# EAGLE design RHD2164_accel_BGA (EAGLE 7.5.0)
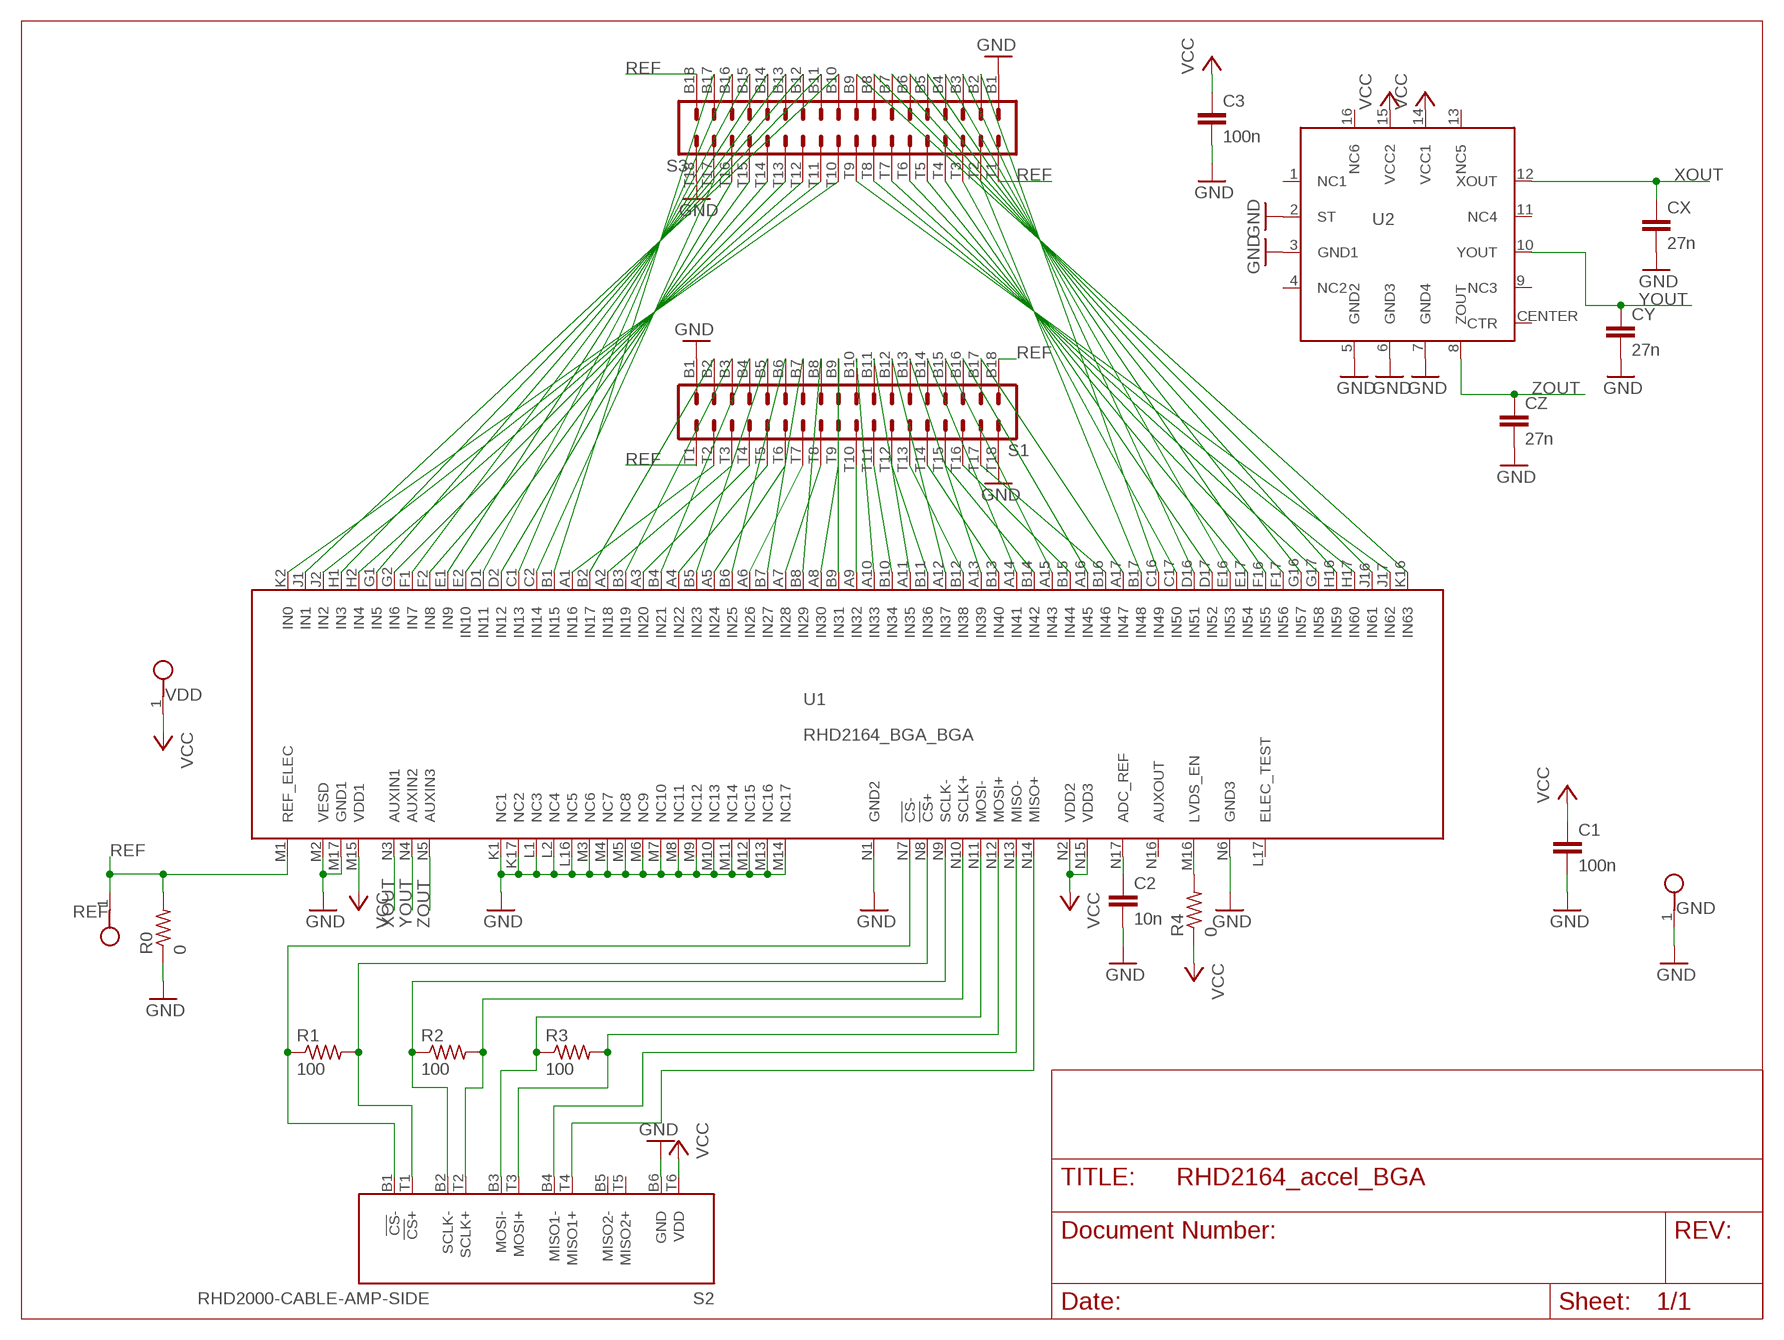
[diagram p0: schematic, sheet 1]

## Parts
C1  100n  C_0402  [0402]
C2  10n  C_0201  [0201]
C3  100n  C_0402  [0402]
CX  27n  C_0402  [0402]
CY  27n  C_0402  [0402]
CZ  27n  C_0402  [0402]
GND  TESTPOINT_SMALL  [TESTPOINT_SMALL]
R0  0  R_0402  [0402]
R1  100  R_0201  [0201]
R2  100  R_0201  [0201]
R3  100  R_0201  [0201]
R4  0  R_0402  [0402]
REF  TESTPOINT_SMALL  [TESTPOINT_SMALL]
S1  OMNETICS_A79025  [OMNETICS_A79025]
S2  RHD2000-CABLE-AMP-SIDE  [OMNETICS_PZN-12-AA]
S3  OMNETICS_A79025  [OMNETICS_A79025]
U1  RHD2164_BGA_BGA  [BGA104_9X7]
U2  ADXL335_IDAX  [ADXL335_IDAX]
VDD  TESTPOINT_SMALL  [TESTPOINT_SMALL]

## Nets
GND [thick]: C1.2 C2.2 C3.2 CX.2 CY.2 CZ.2 GND.1 R0.1 S1.B1 S1.T18 S2.B6(GND) S3.B1 S3.T18 U1.K1(NC1) U1.K17(NC2) U1.L1(NC3) U1.L2(NC4) U1.L16(NC5) U1.M2(VESD) U1.M3(NC6) U1.M4(NC7) U1.M5(NC8) U1.M6(NC9) U1.M7(NC10) U1.M8(NC11) U1.M9(NC12) U1.M10(NC13) U1.M11(NC14) U1.M12(NC15) U1.M13(NC16) U1.M14(NC17) U1.M17(GND1) U1.N1(GND2) U1.N6(GND3) U2.2(ST) U2.3(GND1) U2.5(GND2) U2.6(GND3) U2.7(GND4)
N$1: C2.1 U1.N17(ADC_REF)
N$2: S1.T2 U1.A1(IN16)
N$3: S1.B2 U1.B2(IN17)
N$4: S1.T3 U1.A2(IN18)
N$5: S1.B3 U1.B3(IN19)
N$6: S1.T4 U1.A3(IN20)
N$7: S1.B4 U1.B4(IN21)
N$8: S1.T5 U1.A4(IN22)
N$9: S1.B5 U1.B5(IN23)
N$10: S1.T6 U1.A5(IN24)
N$11: R1.1 S2.B1(!CS!-) U1.N7(!CS!-)
N$12: S1.B6 U1.B6(IN25)
N$13: S1.T7 U1.A6(IN26)
N$14: S1.B7 U1.B7(IN27)
N$15: S1.T8 U1.A7(IN28)
N$16: S1.B8 U1.B8(IN29)
N$17: S1.T9 U1.A8(IN30)
N$18: S1.B9 U1.B9(IN31)
N$19: S1.T10 U1.A9(IN32)
N$20: S1.B10 U1.A10(IN33)
N$21: S1.T11 U1.B10(IN34)
N$22: S1.B11 U1.A11(IN35)
N$23: S1.T12 U1.B11(IN36)
N$24: S1.B12 U1.A12(IN37)
N$25: S1.T13 U1.B12(IN38)
N$26: S1.B13 U1.A13(IN39)
N$27: S1.T14 U1.B13(IN40)
N$28: S1.B14 U1.A14(IN41)
N$29: S1.T15 U1.B14(IN42)
N$30: S1.B15 U1.A15(IN43)
N$31: S1.T16 U1.B15(IN44)
N$32: S1.B16 U1.A16(IN45)
N$33: S1.T17 U1.B16(IN46)
N$34: S1.B17 U1.A17(IN47)
N$35: R1.2 S2.T1(!CS!+) U1.N8(!CS!+)
N$36: R2.1 S2.B2(SCLK-) U1.N9(SCLK-)
N$37: R2.2 S2.T2(SCLK+) U1.N10(SCLK+)
N$38: R3.1 S2.B3(MOSI-) U1.N11(MOSI-)
N$39: R3.2 S2.T3(MOSI+) U1.N12(MOSI+)
N$40: S2.B4(MISO1-) U1.N13(MISO-)
N$41: S3.B17 U1.B1(IN15)
N$42: R4.2 U1.M16(LVDS_EN)
N$43: S3.T17 U1.C2(IN14)
N$44: S3.B16 U1.C1(IN13)
N$45: S3.T16 U1.D2(IN12)
N$46: S3.B15 U1.D1(IN11)
N$47: S3.T15 U1.E2(IN10)
N$48: S3.B14 U1.E1(IN9)
N$49: S3.T14 U1.F2(IN8)
N$50: S3.B13 U1.F1(IN7)
N$51: S3.T13 U1.G2(IN6)
N$52: S3.B12 U1.G1(IN5)
N$53: S3.T12 U1.H2(IN4)
N$54: S3.B11 U1.H1(IN3)
N$55: S3.T11 U1.J2(IN2)
N$56: S3.B10 U1.J1(IN1)
N$57: S3.T10 U1.K2(IN0)
N$58: S3.T2 U1.B17(IN48)
N$59: S3.B2 U1.C16(IN49)
N$60: S3.T3 U1.C17(IN50)
N$61: S3.B3 U1.D16(IN51)
N$62: S3.T4 U1.D17(IN52)
N$63: S3.B4 U1.E16(IN53)
N$64: S3.T5 U1.E17(IN54)
N$65: S3.B5 U1.F16(IN55)
N$66: S3.T6 U1.F17(IN56)
N$67: S3.B6 U1.G16(IN57)
N$68: S3.T7 U1.G17(IN58)
N$69: S3.B7 U1.H16(IN59)
N$70: S3.T8 U1.H17(IN60)
N$71: S3.B8 U1.J16(IN61)
N$72: S3.T9 U1.J17(IN62)
N$73: S3.B9 U1.K16(IN63)
N$74: S2.T4(MISO1+) U1.N14(MISO+)
REF [thick]: R0.2 REF.1 S1.B18 S1.T1 S3.B18 S3.T1 U1.M1(REF_ELEC)
VCC [thick]: C1.1 C3.1 R4.1 S2.T6(VDD) U1.M15(VDD1) U1.N2(VDD2) U1.N15(VDD3) U2.14(VCC1) U2.15(VCC2) VDD.1
XOUT: CX.1 U1.N3(AUXIN1) U2.12(XOUT)
YOUT: CY.1 U1.N4(AUXIN2) U2.10(YOUT)
ZOUT: CZ.1 U1.N5(AUXIN3) U2.8(ZOUT)
Unconnected: S2.B5(MISO2-) S2.T5(MISO2+) U1.L17(ELEC_TEST) U1.N16(AUXOUT) U2.1(NC1) U2.4(NC2) U2.9(NC3) U2.11(NC4) U2.13(NC5) U2.16(NC6) U2.CENTER(CTR)

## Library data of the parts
C1-C3 CX CY CZ = RHD2000_eval_board:C: Capacitor
GND REF VDD = RHD2000_eval_board:TESTPOINT: PCB Test Point
R0 R1-R4 = RHD2000_eval_board:R: Resistor
S1 S3 = RHD2000:OMNETICS_A79025: Omnetics A79025 36-pin connector
S2 = RHD2000:RHD2000-CABLE-AMP-SIDE: Omnetics A79623 PZN-12-AA connector for SPI interface (amplifier side)
U1 = INTAN:RHD2164_BGA: Intan Technologies RHD2164 chip, BGA package (9x7mm 104-pin)
U2 = harrison:ADXL335

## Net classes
1 thick: width 0.102 mm
2 power: width 0.61 mm

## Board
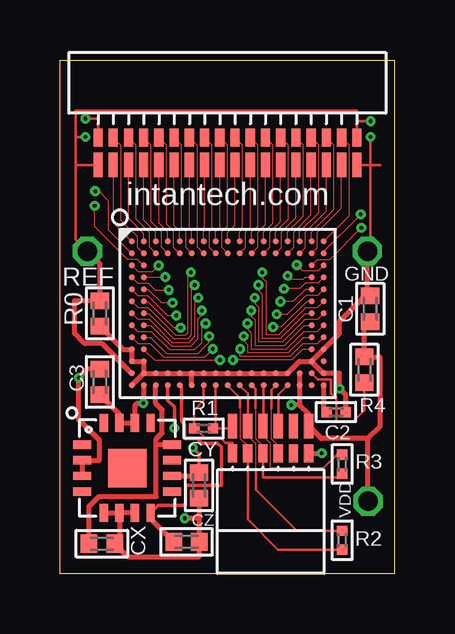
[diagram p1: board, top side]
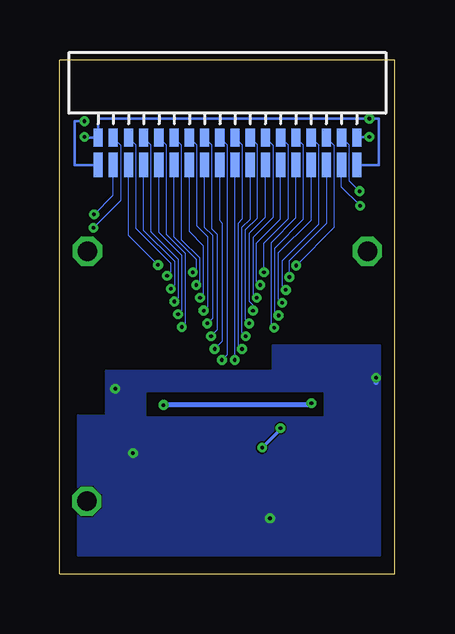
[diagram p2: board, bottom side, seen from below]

Size 13.97 x 21.42 mm. Coordinates in mm from the lower left corner, seen from the top.
Outline: 0,0 0,21.43 13.97,21.43 13.97,0 0,0
Copper layers (1*16): Top 0.035mm / dielectric 1.5mm / Bottom 0.035mm
Design rules "default *": minimum track width 2mil, minimum drill 6mil, track to track 2mil, track to pad 2mil, pad to pad 2mil, via to via 2mil, smd to smd 2mil, copper to edge 20mil, drill to drill 15mil, minimum pad ring 5mil, minimum via ring 5mil, stop-mask expansion 2mil, vias tented up to drill 0mil, thermal gap 10mil

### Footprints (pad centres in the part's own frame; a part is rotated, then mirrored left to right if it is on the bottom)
0402 = smd 0.686 x 0.762: 1 -0.533,0; 2 0.533,0
0201 = smd 0.432 x 0.432: 1 -0.394,0; 2 0.394,0
TESTPOINT_SMALL = drill 0.813 octagon: 1 0,0
OMNETICS_A79025 = smd 0.381 x 0.762: B1 -5.397,-1.016; B2 -4.763,-1.016; B3 -4.128,-1.016; B4 -3.493,-1.016; B5 -2.857,-1.016; B6 -2.223,-1.016; B7 -1.587,-1.016; B8 -0.953,-1.016; B9 -0.318,-1.016; B10 0.318,-1.016; B11 0.953,-1.016; B12 1.587,-1.016; B13 2.223,-1.016; B14 2.857,-1.016; B15 3.493,-1.016; B16 4.128,-1.016; B17 4.763,-1.016; B18 5.397,-1.016 | smd 0.381 x 1.016: T1 -5.397,-2.159; T2 -4.763,-2.159; T3 -4.128,-2.159; T4 -3.493,-2.159; T5 -2.857,-2.159; T6 -2.223,-2.159; T7 -1.587,-2.159; T8 -0.953,-2.159; T9 -0.318,-2.159; T10 0.318,-2.159; T11 0.953,-2.159; T12 1.587,-2.159; T13 2.223,-2.159; T14 2.857,-2.159; T15 3.493,-2.159; T16 4.128,-2.159; T17 4.763,-2.159; T18 5.397,-2.159
OMNETICS_PZN-12-AA = smd 0.381 x 0.762: B1 1.587,-1.016; B2 0.953,-1.016; B3 0.318,-1.016; B4 -0.318,-1.016; B5 -0.953,-1.016; B6 -1.587,-1.016 | smd 0.381 x 1.016: T1 1.587,-2.159; T2 0.953,-2.159; T3 0.318,-2.159; T4 -0.318,-2.159; T5 -0.953,-2.159; T6 -1.587,-2.159
BGA104_9X7 = smd 0.25 x 0.25: A1 -4,3; A2 -3.5,3; A3 -3,3; A4 -2.5,3; A5 -2,3; A6 -1.5,3; A7 -1,3; A8 -0.5,3; A9 0,3; A10 0.5,3; A11 1,3; A12 1.5,3; A13 2,3; A14 2.5,3; A15 3,3; A16 3.5,3; A17 4,3; B1 -4,2.5; B2 -3.5,2.5; B3 -3,2.5; B4 -2.5,2.5; B5 -2,2.5; B6 -1.5,2.5; B7 -1,2.5; B8 -0.5,2.5; B9 0,2.5; B10 0.5,2.5; B11 1,2.5; B12 1.5,2.5; B13 2,2.5; B14 2.5,2.5; B15 3,2.5; B16 3.5,2.5; B17 4,2.5; C1 -4,2; C2 -3.5,2; C16 3.5,2; C17 4,2; D1 -4,1.5; D2 -3.5,1.5; D16 3.5,1.5; D17 4,1.5; E1 -4,1; E2 -3.5,1; E16 3.5,1; E17 4,1; F1 -4,0.5; F2 -3.5,0.5; F16 3.5,0.5; F17 4,0.5; G1 -4,0; G2 -3.5,0; G16 3.5,0; G17 4,0; H1 -4,-0.5; H2 -3.5,-0.5; H16 3.5,-0.5; H17 4,-0.5; J1 -4,-1; J2 -3.5,-1; J16 3.5,-1; J17 4,-1; K1 -4,-1.5; K2 -3.5,-1.5; K16 3.5,-1.5; K17 4,-1.5; L1 -4,-2; L2 -3.5,-2; L16 3.5,-2; L17 4,-2; M1 -4,-2.5; M2 -3.5,-2.5; M3 -3,-2.5; M4 -2.5,-2.5; M5 -2,-2.5; M6 -1.5,-2.5; M7 -1,-2.5; M8 -0.5,-2.5; M9 0,-2.5; M10 0.5,-2.5; M11 1,-2.5; M12 1.5,-2.5; M13 2,-2.5; M14 2.5,-2.5; M15 3,-2.5; M16 3.5,-2.5; M17 4,-2.5; N1 -4,-3; N2 -3.5,-3; N3 -3,-3; N4 -2.5,-3; N5 -2,-3; N6 -1.5,-3; N7 -1,-3; N8 -0.5,-3; N9 0,-3; N10 0.5,-3; N11 1,-3; N12 1.5,-3; N13 2,-3; N14 2.5,-3; N15 3,-3; N16 3.5,-3; N17 4,-3
ADXL335_IDAX = smd 0.75 x 0.35: 1 -1.875,0.975; 2 -1.875,0.325; 3 -1.875,-0.325; 4 -1.875,-0.975; 9 1.875,-0.975; 10 1.875,-0.325; 11 1.875,0.325; 12 1.875,0.975 | smd 0.35 x 0.75: 5 -0.975,-1.875; 6 -0.325,-1.875; 7 0.325,-1.875; 8 0.975,-1.875; 13 0.975,1.875; 14 0.325,1.875; 15 -0.325,1.875; 16 -0.975,1.875 | smd 1.6 x 1.6: CENTER 0,0

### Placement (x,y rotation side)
C1  12.94,11.05 90 top
C2  11.52,6.74 0 top
C3  1.67,8 90 top
CX  1.75,1.25 0 top
CY  5.8,3.68 270 top
CZ  5.28,1.33 0 top
GND  12.83,13.45 0 top
R0  1.66,10.86 90 top
R1  5.99,6.06 0 top
R2  11.77,1.4 90 top
R3  11.77,4.57 90 top
R4  12.7,8.51 270 top
REF  1.14,13.45 0 top
S1  6.99,19.2 0 top
S2  8.79,4 180 top
S3  6.99,19.2 0 bottom
U1  7,10.86 0 top
U2  2.8,4.41 0 top
VDD  12.85,3.02 0 top

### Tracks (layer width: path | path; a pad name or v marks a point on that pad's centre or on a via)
GND  (via drill 0.15)
  Top 0.102: 13.36,17.04 12.95,17.04 | v1.07,18.97 1.59,18.97 S1.B1 | S1.T18 12.95,17.04 | 12.95,17.04 v12.95,18.21 | 12.95,17.04 12.95,13.58 GND.1
  Top 0.203: U1.N1 U1.M2 | U1.M2 U1.L2 U1.L1 U1.K1 2.63,9.36 R0.1 | U1.M2 U1.M3 U1.M4 U1.M5 U1.M6 | U1.N6 U1.M6 | U1.M6 U1.M7 U1.M8 U1.M9 U1.M10 U1.M11 U1.M12 U1.M13 U1.M14 10,8.86 U1.L16 | U1.L16 U1.M17 | U1.L16 U1.K17 11.66,10.02 11.66,10.52 12.72,11.58 C1.2 | U1.M17 11.1,8.36 | S2.B6 10.91,5.02 v10.92,5.03 | C3.2 1.14,8.53 v0.79,8.18 0.79,6.43 1.65,5.56 1.65,4.73 U2.2 U2.3 | CY.2 5.8,2.31 v5.21,2.31 5.82,2.31 CZ.2 5.82,0.71 2.83,0.71 CX.2 2.48,1.45 U2.6 | U2.5 U2.6 | U2.7 U2.6 | U1.M17 11.66,8.36 v11.66,7.72 11.91,7.47 C2.2 | C1.2 12.83,11.44 | C1.2 12.83,11.7 GND.1
  Bottom 0.102: S3.T18 0.66,17.04 0.66,18.97 v1.07,18.97 12.38,18.97 S3.B1 12.95,18.19 v12.95,18.21
  Bottom 0.203: v10.92,5.03 11.02,5.03 | v0.79,8.18 0.79,7.98 | v5.21,2.31 5.08,2.31
  pour Bottom: 2.92,6.53 10.41,6.53 10.41,0.76 2.92,0.76
  pour Bottom: 0.64,0.76 0.64,9.53 5.08,9.53 5.08,8.46 12.04,8.46 12.04,6.58 13.21,6.6 13.21,0.76 10.41,0.76 10.41,7.62 2.92,7.62 2.92,0.76
N$1
  Top 0.203: U1.N17 11,6.87 C2.1
N$2
  Top 0.051: S1.T2 2.22,14.63 U1.A1
N$3
  Top 0.051: S1.B2 2.54,17.87 2.54,14.76 3.23,14.07 3.23,13.63 U1.B2
N$4
  Top 0.051: U1.A2 3.5,14.18 2.86,14.82 S1.T3
N$5
  Top 0.051: U1.B3 3.73,13.62 3.73,14.22 3.17,14.78 3.17,17.87 S1.B3
N$6
  Top 0.051: U1.A3 4,14.24 3.49,14.74 S1.T4
N$7
  Top 0.051: U1.B4 4.24,13.61 4.24,14.25 3.81,14.68 3.81,17.87 S1.B4
N$8
  Top 0.051: U1.A4 4.5,14.25 4.13,14.62 S1.T5
N$9
  Top 0.051: U1.B5 4.75,13.61 4.75,14.28 4.45,14.58 4.45,17.87 S1.B5
N$10
  Top 0.051: U1.A5 5,14.28 4.76,14.52 S1.T6
N$11
  Top 0.102: U1.N7 6,7.22 5.6,6.82 R1.1 5.65,6.06 6.04,5.66 6.71,5.66 6.91,5.46 7.2,5.46 S2.B1 7.2,5.14
N$12
  Top 0.051: U1.B6 5.26,13.6 5.26,14.28 5.08,14.45 5.08,17.87 S1.B6
N$13
  Top 0.051: U1.A6 5.5,14.29 5.4,14.39 S1.T7
N$14
  Top 0.051: U1.B7 5.74,13.62 5.74,17.84 S1.B7
N$15
  Top 0.051: U1.A7 6,14.28 6.03,14.31 S1.T8
N$16
  Top 0.051: U1.B8 6.25,13.61 6.25,14.28 6.35,14.38 6.35,17.87 S1.B8
N$17
  Top 0.051: U1.A8 6.5,14.27 6.67,14.44 S1.T9
N$18
  Top 0.051: U1.B9 6.76,13.6 6.76,14.28 6.99,14.5 6.99,17.87 S1.B9
N$19
  Top 0.051: U1.A9 7,14.24 7.3,14.54 S1.T10
N$20
  Top 0.051: U1.A10 7.5,14.25 7.62,14.38 7.62,17.87 S1.B10
N$21
  Top 0.051: U1.B10 7.75,13.61 7.75,14.25 7.94,14.44 S1.T11
N$22
  Top 0.051: U1.A11 8,14.25 8.26,14.5 8.26,17.87 S1.B11
N$23
  Top 0.051: U1.B11 8.26,13.62 8.26,14.25 8.57,14.57 S1.T12
N$24
  Top 0.051: U1.A12 8.5,14.24 8.89,14.63 8.89,17.87 S1.B12
N$25
  Top 0.051: U1.B12 8.76,13.62 8.76,14.25 9.21,14.69 S1.T13
N$26
  Top 0.051: U1.A13 9,14.26 9.53,14.78 9.53,17.87 S1.B13
N$27
  Top 0.051: U1.B13 9.25,13.61 9.25,14.25 9.84,14.85 S1.T14
N$28
  Top 0.051: U1.A14 9.5,14.25 10.16,14.91 10.16,17.87 S1.B14
N$29
  Top 0.051: U1.B14 9.75,13.61 9.75,14.25 10.48,14.97 S1.T15
N$30
  Top 0.051: U1.A15 10,14.27 10.79,15.06 10.79,17.87 S1.B15
N$31
  Top 0.051: U1.B15 10.24,13.6 10.24,14.25 11.11,15.13 S1.T16
N$32
  Top 0.051: U1.A16 10.5,14.26 11.43,15.19 11.43,17.87 S1.B16
N$33
  Top 0.051: U1.B16 10.74,13.61 10.74,14.25 11.75,15.25 S1.T17
N$34
  Top 0.051: S1.B17 12.06,17.87 12.06,14.93 U1.A17
N$35
  Top 0.102: 7.2,6.14 S2.T1 7.2,6.06 R1.2 6.5,6.06 U1.N8
N$36
  Top 0.051: 7.52,6.93 7.52,5.64 7.84,5.32 S2.B2
  Top 0.102: U1.N9 7.52,7.34 7.52,6.93 | S2.B2 7.84,2.26 9.09,1 R2.1
N$37
  Top 0.051: 8.18,4.37 8.18,5.41 7.84,5.75 S2.T2
  Top 0.102: U1.N10 7.84,7.52 S2.T2 | 8.18,4.37 8.18,3.5 9.89,1.79 R2.2
N$38
  Top 0.051: 8.15,6.91 8.15,5.64 8.47,5.32 S2.B3
  Top 0.102: U1.N11 8.15,7.7 8.15,6.91 | R3.1 11.61,4.01 8.48,4.01 8.47,4.03 S2.B3
N$39
  Top 0.051: 8.79,4.39 8.79,5.44 8.47,5.75 S2.T3
  Top 0.102: U1.N12 8.5,6.19 S2.T3 | R3.2 11.54,4.97 10.97,4.39 8.79,4.39
N$40
  Top 0.051: S2.B4 9.11,5.32 8.81,5.61 8.81,6.88
  Top 0.102: 8.81,6.88 8.81,7.67 U1.N13
N$41  (via drill 0.15)
  Top 0.051: v1.47,15.95 1.63,15.95 2.03,15.54 2.03,14.32 U1.B1
  Bottom 0.051: v1.47,15.95 1.91,16.38 1.91,17.87 S3.B17
N$42
  Top 0.102: U1.M16 10.75,8.1 11.3,8.1 11.3,7.52 11.53,7.29 11.53,6.33 12.22,6.33 12.7,6.81 R4.2
N$43  (via drill 0.15)
  Top 0.051: U1.C2 3.25,13.11 2.82,13.11 1.45,14.48 v1.45,15.34
  Bottom 0.051: v1.45,15.34 2.22,16.12 S3.T17
N$44  (via drill 0.15)
  Top 0.051: U1.C1 3.26,12.6 3.86,12.6 v4.12,12.85
  Bottom 0.051: S3.B16 2.54,17.87 2.54,14.43 v4.12,12.85
N$45  (via drill 0.15)
  Top 0.051: U1.D2 3.51,12.34 3.54,12.37 v4.39,12.37
  Bottom 0.051: S3.T16 2.86,14.59 4.42,13.03 4.42,12.39 v4.39,12.37
N$46  (via drill 0.15)
  Top 0.051: U1.D1 3.24,12.12 3.68,12.12 3.96,11.84 v4.55,11.84
  Bottom 0.051: S3.B15 3.17,17.87 3.17,14.58 4.7,13.06 4.7,11.99 v4.55,11.84
N$47  (via drill 0.15)
  Top 0.051: U1.E2 3.69,11.86 4.24,11.3 v4.7,11.3
  Bottom 0.051: S3.T15 3.48,14.76 4.85,13.39 4.85,11.46 v4.7,11.3
N$48  (via drill 0.15)
  Top 0.051: U1.E1 3.25,11.61 3.66,11.61 4.5,10.77 v4.85,10.77
  Bottom 0.051: S3.B14 3.81,17.87 3.81,14.78 5,13.59 5,10.92 v4.85,10.77
N$49  (via drill 0.15)
  Top 0.051: U1.F2 3.65,11.36 4.75,10.26 v5.03,10.26
  Bottom 0.051: v5.03,10.26 5.16,10.39 5.16,13.82 4.13,14.85 S3.T14
N$50  (via drill 0.15)
  Top 0.051: U1.F1 3.26,11.1 3.68,11.1 4.83,9.96 5.23,9.96 5.33,10.06 5.33,12.45 v5.46,12.57
  Bottom 0.051: S3.B13 4.45,17.87 4.45,14.81 5.46,13.79 v5.46,12.57
N$51  (via drill 0.15)
  Top 0.051: U1.G2 3.7,10.86 4.75,9.8 5.33,9.8 5.49,9.96 5.49,11.91 v5.61,12.04
  Bottom 0.051: v5.61,12.04 5.77,12.19 5.77,13.79 4.76,14.8 S3.T13
N$52  (via drill 0.15)
  Top 0.051: U1.G1 3.24,10.62 3.71,10.62 4.67,9.65 5.38,9.65 5.64,9.91 5.64,11.38 v5.77,11.51
  Bottom 0.051: S3.B12 5.08,17.87 5.08,14.86 5.92,14.02 5.92,11.66 v5.77,11.51
N$53  (via drill 0.15)
  Top 0.051: U1.H2 3.79,10.36 4.65,9.5 5.46,9.5 5.77,9.8 5.77,10.64 5.92,10.79 v5.92,10.97
  Bottom 0.051: v5.92,10.97 5.92,11.2 6.07,11.35 6.07,14.2 5.4,14.87 S3.T12
N$54  (via drill 0.15)
  Top 0.051: U1.H1 3.25,10.11 3.81,10.11 4.57,9.35 5.61,9.35 5.92,9.65 5.92,10.29 v6.07,10.44
  Bottom 0.051: S3.B11 5.74,17.89 5.74,14.83 6.22,14.35 6.22,10.59 v6.07,10.44
N$55  (via drill 0.15)
  Top 0.051: U1.J2 3.78,9.86 4.45,9.2 5.77,9.2 6.22,9.65 v6.22,9.91
  Bottom 0.051: v6.22,9.91 6.38,10.06 6.38,14.45 6.03,14.8 S3.T11
N$56  (via drill 0.15)
  Top 0.051: U1.J1 3.25,9.6 3.76,9.6 4.32,9.04 6.04,9.04 v6.38,9.37
  Bottom 0.051: S3.B10 6.35,17.87 6.35,14.81 6.53,14.63 6.53,9.53 v6.38,9.37
N$57  (via drill 0.15)
  Top 0.051: U1.K2 3.94,8.91 v6.68,8.91
  Bottom 0.051: v6.68,8.91 6.67,8.93 S3.T10
N$58  (via drill 0.15)
  Top 0.051: U1.B17 11,13.44 v12.55,14.99
  Bottom 0.051: 11.75,16.62 S3.T2 11.75,15.79 v12.55,14.99
N$59  (via drill 0.15)
  Top 0.051: U1.C16 10.75,13.11 11.25,13.11 v12.57,14.43
  Bottom 0.051: S3.B2 11.43,17.87 11.43,15.57 v12.57,14.43
N$60  (via drill 0.15)
  Top 0.051: U1.C17 10.76,12.62 10.13,12.62 v9.88,12.88
  Bottom 0.051: S3.T3 11.11,14.11 v9.88,12.88
N$61  (via drill 0.15)
  Top 0.051: U1.D16 10.22,12.36 10.13,12.27 9.65,12.27 v9.5,12.42
  Bottom 0.051: S3.B3 10.79,17.87 10.79,14.4 9.35,12.95 9.35,12.57 v9.5,12.42
N$62  (via drill 0.15)
  Top 0.051: U1.D17 10.76,12.12 10.24,12.12 10.01,11.89 v9.35,11.89
  Bottom 0.051: S3.T4 10.48,14.31 9.2,13.03 9.2,12.04 v9.35,11.89
N$63  (via drill 0.15)
  Top 0.051: U1.E16 10.23,11.86 9.73,11.35 v9.2,11.35
  Bottom 0.051: S3.B4 10.16,17.87 10.16,14.25 9.04,13.13 9.04,11.51 v9.2,11.35
N$64  (via drill 0.15)
  Top 0.051: U1.E17 10.75,11.61 10.26,11.61 9.47,10.82 v9.04,10.82
  Bottom 0.051: S3.T5 9.84,14.24 8.89,13.28 8.89,10.97 v9.04,10.82
N$65  (via drill 0.15)
  Top 0.051: U1.F16 10.29,11.36 9.22,10.29 v8.89,10.29
  Bottom 0.051: S3.B5 9.53,17.87 9.53,14.15 8.74,13.36 8.74,10.44 v8.89,10.29
N$66  (via drill 0.15)
  Top 0.051: v8.43,12.57 8.43,12.34 8.59,12.19 8.59,9.98 9.14,9.98 10.26,11.1 10.74,11.1 U1.F17
  Bottom 0.051: S3.T6 9.21,14.03 8.28,13.11 8.28,12.72 v8.43,12.57
N$67  (via drill 0.15)
  Top 0.051: v8.28,12.04 8.28,11.81 8.43,11.66 8.43,9.83 9.22,9.83 10.25,10.86 U1.G16
  Bottom 0.051: S3.B6 8.89,17.87 8.89,13.92 8.13,13.16 8.13,12.19 v8.28,12.04
N$68  (via drill 0.15)
  Top 0.051: v8.13,11.51 8.13,11.28 8.28,11.12 8.28,9.68 9.3,9.68 10.24,10.62 10.76,10.62 U1.G17
  Bottom 0.051: v8.13,11.51 7.98,11.66 7.98,13.66 8.57,14.26 S3.T7
N$69  (via drill 0.15)
  Top 0.051: v7.98,10.97 7.98,10.74 8.13,10.59 8.13,9.53 9.37,9.53 10.21,10.36 U1.H16
  Bottom 0.051: v7.98,10.97 7.8,11.15 7.8,14.05 8.26,14.5 8.26,17.87 S3.B7
N$70  (via drill 0.15)
  Top 0.051: v7.82,10.44 7.82,10.21 7.98,10.06 7.98,9.37 9.45,9.37 10.19,10.11 10.75,10.11 U1.H17
  Bottom 0.051: v7.82,10.44 7.59,10.67 7.59,14.1 7.94,14.44 S3.T8
N$71  (via drill 0.15)
  Top 0.051: v7.67,9.91 7.67,9.7 7.82,9.55 7.82,9.22 9.53,9.22 10.16,9.86 U1.J16
  Bottom 0.051: v7.67,9.91 7.39,10.19 7.39,14.15 7.62,14.38 7.62,17.87 S3.B8
N$72  (via drill 0.15)
  Top 0.051: v7.52,9.37 7.52,9.07 9.6,9.07 10.13,9.6 10.74,9.6 U1.J17
  Bottom 0.051: S3.T9 7.3,14.72 7.19,14.61 7.19,9.7 v7.52,9.37
N$73  (via drill 0.15)
  Top 0.051: U1.K16 10.12,9.36 9.68,8.91 v7.21,8.91
  Bottom 0.051: S3.B9 6.99,17.87 6.99,9.14 v7.21,8.91
N$74
  Top 0.102: U1.N14 9.11,7.47 S2.T4
REF  (via drill 0.15)
  Top 0.102: 12.38,18.87 S1.B18 | v12.95,18.87 12.38,18.87 | 0.66,17.04 0.66,18.21 | 0.66,18.21 v1.07,18.21 | 0.66,18.21 0.66,19.3 12.38,19.3 12.38,18.87 | S1.T1 0.66,17.04 | 0.66,17.04 0.66,13.93 REF.1
  Top 0.203: REF.1 1.66,12.93 R0.2 0.61,11.39 0.61,10.03 1.04,9.6 1.75,9.6 U1.M1
  Bottom 0.102: v12.95,18.87 13.36,18.87 13.36,17.04 S3.T1 | S3.B18 1.59,18.21 v1.07,18.21
VCC  (via drill 0.15)
  Top 0.203: U1.M15 U1.N15 10,7.04 | 10,7.04 v9.65,7.04 | 10,7.04 10.38,6.66 S2.T6 | 10.38,6.02 S2.T6 | C3.1 2.48,6.65 U2.15 U2.14 3.13,7.02 3.23,7.11 v3.48,7.11 3.5,7.13 U1.N2 | VDD.1 12.85,5.64 | 12.85,5.64 10.9,5.64 S2.T6 | 12.85,5.64 13.34,6.12 13.34,9.04 R4.1 12.7,10.27 C1.1
  Bottom 0.203: v9.65,7.04 3.56,7.04 v3.48,7.11
XOUT
  Top 0.203: CX.1 1.22,2.82 1.63,3.23 4.01,3.23 4.01,5.38 | 4.01,5.38 U2.12 | 4.01,5.38 4.01,5.61 4.27,5.87 4.27,6.83 4,7.1 U1.N3
YOUT  (via drill 0.15)
  Top 0.102: U2.10 5.8,4.08 CY.1
  Top 0.152: U1.N4 4.5,7.24 4.78,6.96 v4.78,6.07 | CY.1 5.8,4.99 v5.54,5.26
  Top 0.203: U2.10 5.59,4.08
  Bottom 0.152: v4.78,6.07 4.78,6.02 v5.54,5.26
ZOUT
  Top 0.152: U2.8 4.09,2.85 5.23,2.85 5.23,3.68 6.73,3.68 6.73,5.28 6.58,5.44 5.92,5.44 5.71,5.64 5.21,5.64 5.21,6.22 5.08,6.35 5.08,7.78 U1.N5
  Top 0.203: CZ.1 3.78,2.3 U2.8

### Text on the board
tPlace: intantech.com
